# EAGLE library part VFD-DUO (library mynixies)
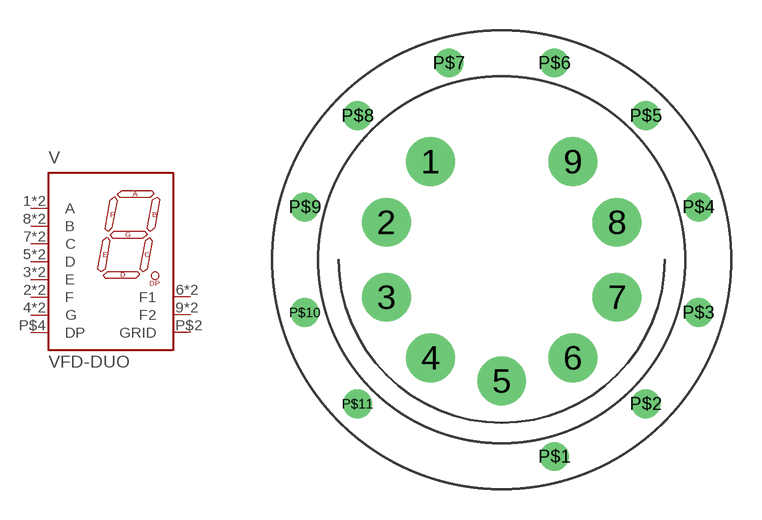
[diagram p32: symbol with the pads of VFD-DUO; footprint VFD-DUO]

Designator prefix V

## VFD-DUO  [VFD-DUO]
1  A  pas
2  F  pas
3  E  pas
4  G  pas
5  D  pas
6  F1  pas
7  C  pas
8  B  pas
9  F2  pas
P$1  F2  pas
P$2  GRID  pas
P$3  C  pas
P$4  DP  pas
P$5  B  pas
P$6  A  pas
P$7  G  pas
P$8  F  pas
P$9  E  pas
P$10  D  pas
P$11  F1  pas

## Footprint VFD-DUO (pad centres in mm)
drill 1.6: 1 -3.497,4.814; 2 -5.659,1.839; 3 -5.659,-1.839; 4 -3.497,-4.814; 5 0,-5.95; 6 3.497,-4.814; 7 5.659,-1.839; 8 5.659,1.839; 9 3.497,4.814
drill 0.9: P$1 2.588,-9.659; P$2 7.071,-7.071; P$3 9.659,-2.588; P$4 9.659,2.588; P$5 7.071,7.071; P$6 2.588,9.659; P$7 -2.588,9.659; P$8 -7.071,7.071; P$9 -9.659,2.588; P$10 -9.659,-2.588; P$11 -7.071,-7.071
